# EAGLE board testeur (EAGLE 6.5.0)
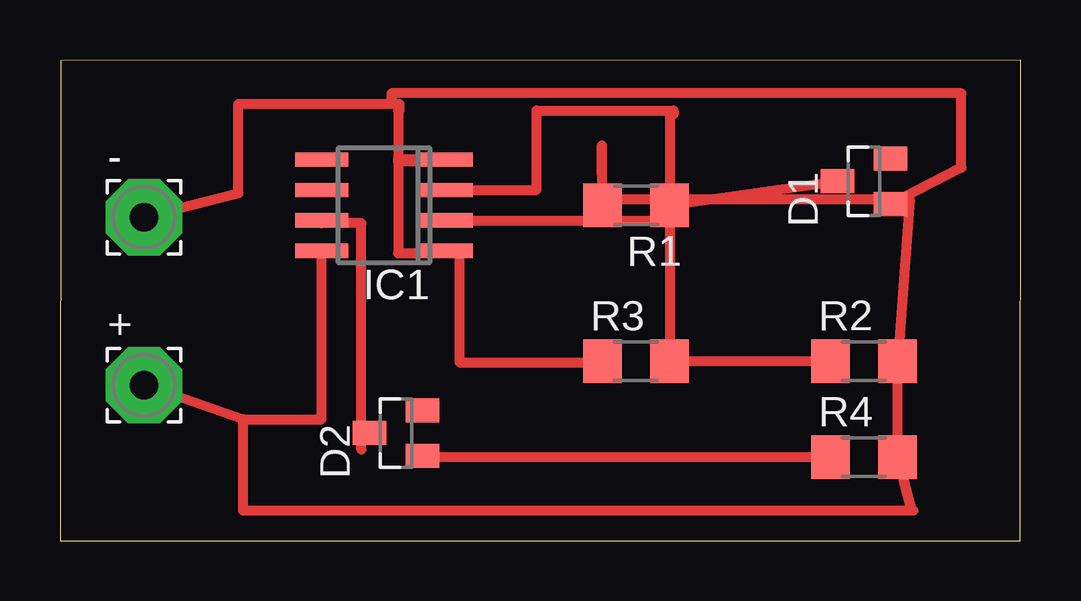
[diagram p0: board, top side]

Size 40.03 x 20.06 mm. Coordinates in mm from the lower left corner, seen from the top.
Outline: 0,0 40.01,0 40.03,20.06 0.03,20.03 0,0
Copper layers (1*16): Top 0.035mm / dielectric 1.5mm / Bottom 0.035mm
Design rules "testeur": minimum track width 10mil, minimum drill 24mil, track to track 0.205mm, track to pad 0.205mm, pad to pad 0.205mm, via to via 0.205mm, smd to smd 8mil, copper to edge 40mil, drill to drill 8mil, minimum pad ring 10mil, minimum via ring 8mil, stop-mask expansion 4mil, vias tented up to drill 0mil, thermal gap 10mil
Net classes: 0 default: clearance 0.205 mm

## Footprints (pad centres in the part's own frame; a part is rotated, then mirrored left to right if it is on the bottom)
3,17/1,2 = drill 1.194 pad 3.175 octagon: 1 0,0
SOT23 = smd 1 x 1.4: 1 -0.95,-1.1; 2 0.95,-1.1; 3 0,1.1
SO08 = smd 0.6 x 2.2: 1 -1.905,-2.6; 2 -0.635,-2.6; 3 0.635,-2.6; 4 1.905,-2.6; 5 1.905,2.6; 6 0.635,2.6; 7 -0.635,2.6; 8 -1.905,2.6
R3216 = smd 1.6 x 1.8: 1 -1.4,0; 2 1.4,0

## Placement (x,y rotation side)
+  WIREPAD3,17/1,2  [3,17/1,2]  3.5,6.5 0 top
-  WIREPAD3,17/1,2  [3,17/1,2]  3.5,13.5 0 top
D1  BZX84C3V3  [SOT23]  33.5,15 90 top
D2  BZX84C3V3  [SOT23]  14,4.5 90 top
IC1  LM311D  [SO08]  13.5,14 90 top
R1  1K  [R3216]  24,14 180 top
R2  10K  [R3216]  33.5,7.5 0 top
R3  8,2K  [R3216]  24,7.5 0 top
R4  330  [R3216]  33.5,3.5 0 top

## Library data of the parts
+ - = wirepad
D1 D2 = diode
IC1 = linear
R1-R4 = eagle-ltspice; SPICEMODEL: NONE; SPICEPREFIX: R

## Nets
N$1: R4.1
N$2: +.1 IC1.8 R1.2 R2.2 R4.2
N$3: IC1.2 R2.1 R3.2
N$4: D1.3 IC1.3 R1.1
N$5: -.1 D1.1 IC1.1 IC1.4 R3.1
N$7: IC1.7

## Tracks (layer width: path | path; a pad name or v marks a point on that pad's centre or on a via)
N$1
  Top 0.406: 14.92,3.5 R4.1
N$2
  Top 0.406: 7.62,5.08 +.1 | 7.62,5.08 7.62,1.27 35.48,1.27 | 35.56,1.27 35.48,1.27 | 35.48,1.27 R4.2 R2.2 35.4,14.25 22.58,14.25 22.58,16.5 R1.2 | 7.62,5.08 10.9,5.08 IC1.8
N$3
  Top 0.406: R2.1 R3.2 25.4,13.37 IC1.2
N$4
  Top 0.406: D1.3 R1.1 25.4,17.78 25.57,17.78 25.57,17.95 19.86,17.95 19.86,14.63 IC1.3
N$5
  Top 0.406: -.1 7.43,14.5 7.43,18.23 13.81,18.23 | 13.81,18.23 14.14,18.23 14.14,17.95 14.09,17.95 14.09,15.84 16.1,15.84 IC1.4 14.09,15.9 14.09,12 16.1,12 IC1.1 16.64,12.1 16.64,7.45 22.6,7.45 R3.1 | D1.1 37.5,15.55 37.5,15.56 37.55,15.56 37.55,18.67 13.81,18.67 13.81,18.23
N$7
  Top 0.406: 12.56,3.81 12.56,13.25 10.9,13.25 IC1.7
